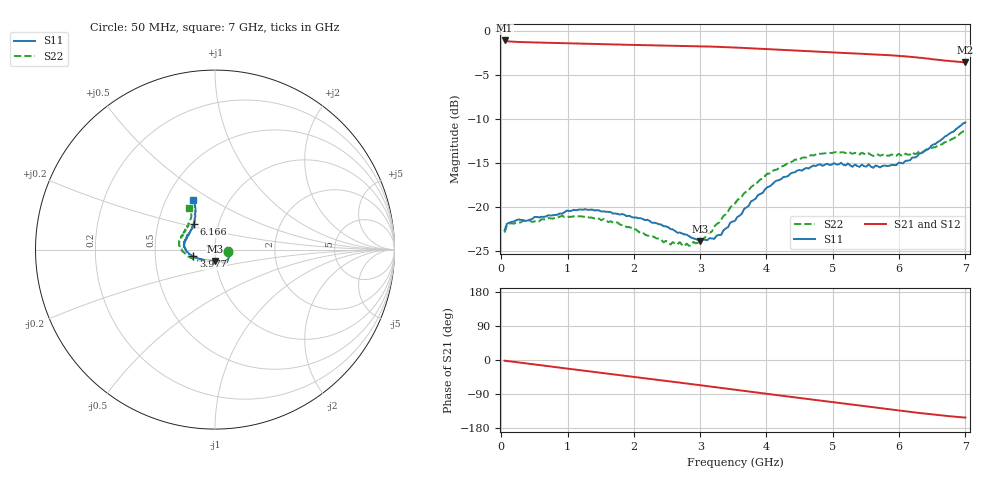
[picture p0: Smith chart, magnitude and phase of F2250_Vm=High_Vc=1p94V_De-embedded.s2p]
! Integrated Device Technology
! Corporate Headquarters
! 6024 Silver Creek Valley Road
! San Jose, CA 95138  USA
! Phone:  1-408-284-8200
! Toll Free:  1-800-223-1366
! Webpage:  http://www.idt.com/
! Timing and RF Division
! 515 Groton Road, Suite 102
! Westford, MA 01886-6024
! Device:  F2250
! Description: Voltage Variable RF Attenuator
! Frequency:  50.0 -  6000.00 MHz
! Package:  3x3 mm Thin QFN Plastic Package: 16 pin
! Ports:  2 RF, 3 DC
!  Pin  1  = GND
!  Pin  2  = NC
!  Pin  3  = RF1  = Port 1
!  Pin  4  = NC
!  Pin  5  = GND
!  Pin  6  = GND
!  Pin  7  = GND
!  Pin  8  = GND
!  Pin  9  = NC
!  Pin 10  = RF2  = Port 2
!  Pin 11  = NC
!  Pin 12  = GND
!  Pin 13  = GND
!  Pin 14  = VCNTRL
!  Pin 15  = VDD
!  Pin 16  = VMODE
! Vcntrl:  1.940 Volts
! Vmode:  +3.300 Volts
! Vdd:  +3.30  Volts
! Current:  1.321 mA
! Data:  The device was measured on a the F2250 evaluation board which has
!  individual transmission lines to the RF pins.  Data was collected
!  using a calibrated network analyzer.  The evaluation board was
!  de-embedded using a TRL calibration technique.
!  The reference plane is the edge of the package pin.
! Misc:  SN 10
!  Action Tracker AT0258
! Date Measured:  2014-11-26
! Date:  2015-10-15  MJV
! Note:
!  Integrated Device Technology supplies this data as a sample of measured
!  data at the package pin for this product.  Your particular data for this
!  product may vary.
!  Data was taken at 25 degrees C.
!  Integrated Device Technology reserves the right to change this data at anytime.
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# GHz S dB R 50
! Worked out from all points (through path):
!   201 points, 50 MHz to 7 GHz, reference 50 ohm
!   highest |S21| = -1.10 dB at 50 MHz (marker M1); lowest = -3.6 dB at 7 GHz (marker M2)
!   group delay of S21, straight-line fit = 61.1 ps
!   lowest |S11| = -23.9 dB at 3.004 GHz (marker M3), VSWR 1.14, Z = 49.8 - j6.4 ohm
!   |S11| at or under -10 dB: start of sweep to end of sweep
!   |S22| runs from -24.4 to -11.3 dB; largest |S21 - S12| = 0.0019
!   S11 on the Smith chart (normalised r, x): 50 MHz: 1.16, -0.02; 3.977 GHz: 0.78, -0.06; 6.166 GHz: 0.76, +0.23; 7 GHz: 0.68, +0.41
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0.05  -22.65 -7.7  -1.10 -1.8  -1.10 -1.8  -22.88 -8.5
0.08475  -21.89 -7.1  -1.18 -2.5  -1.18 -2.5  -22.04 -7.7
0.1195  -21.77 -7.8  -1.22 -3.3  -1.21 -3.3  -21.86 -7.5
0.6755  -21.03 -30.7  -1.36 -15.7  -1.36 -15.7  -21.39 -33.0
1.2315  -20.29 -48.9  -1.48 -27.9  -1.48 -27.9  -21.08 -55.8
1.75275  -20.75 -55.8  -1.57 -39.1  -1.57 -39.1  -21.73 -64.6
2.37825  -21.95 -57.3  -1.66 -52.7  -1.66 -52.7  -23.53 -70.5
2.44775  -22.16 -59.3  -1.67 -54.2  -1.67 -54.3  -24.00 -73.4
2.7605  -23.09 -68.9  -1.72 -61.2  -1.72 -61.2  -24.42 -87.6
3.00375  -23.87 -87.7  -1.76 -66.7  -1.76 -66.7  -23.63 -107.5
3.1775  -23.56 -101.7  -1.80 -70.6  -1.80 -70.6  -22.74 -121.5
3.3165  -23.13 -119.2  -1.84 -73.8  -1.83 -73.8  -21.40 -131.8
3.4555  -21.74 -132.2  -1.88 -76.9  -1.88 -76.9  -20.01 -140.3
3.525  -21.55 -136.9  -1.90 -78.5  -1.90 -78.5  -19.58 -143.7
3.97675  -17.99 -162.8  -2.07 -88.6  -2.07 -88.7  -16.47 -164.3
4.4285  -16.05 -176.4  -2.25 -98.6  -2.26 -98.6  -14.61 -178.5
4.7065  -15.28 175.9  -2.35 -104.8  -2.35 -104.8  -14.14 175.4
5.054  -15.16 167.5  -2.48 -112.4  -2.48 -112.5  -13.76 167.9
5.85325  -15.31 140.9  -2.78 -129.9  -2.78 -130.0  -14.16 148.7
6.166  -14.68 129.3  -2.95 -136.8  -2.95 -136.9  -14.04 140.2
6.54825  -12.83 119.3  -3.25 -144.6  -3.26 -144.7  -13.20 128.0
7  -10.40 113.7  -3.58 -152.0  -3.59 -152.1  -11.29 121.5
